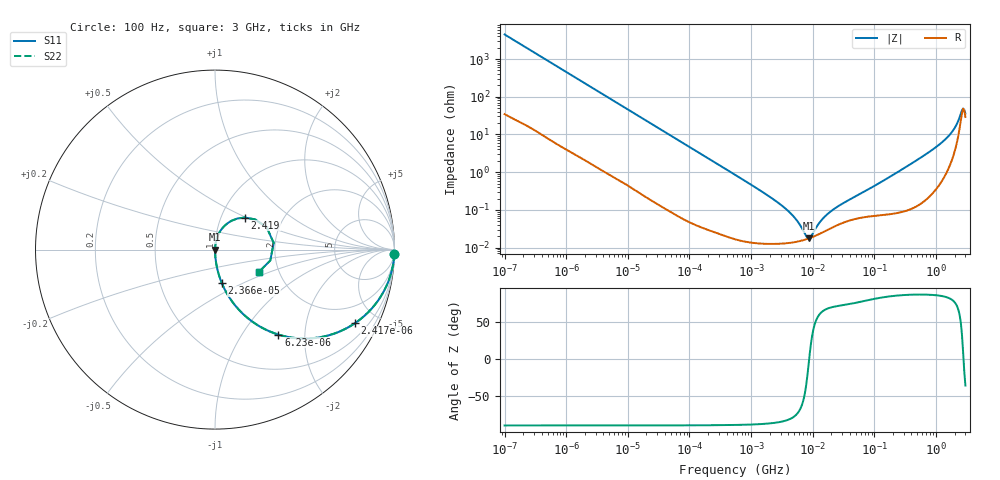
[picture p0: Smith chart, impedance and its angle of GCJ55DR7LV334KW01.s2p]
!Murata Part Number: GCJ55DR7LV334KW01
!These Parameters are Measured in Series Mode Connection
!Data Generated on Mar 13, 2026
!  o--ll--o
!Port1  Port2
!  o------o
!Operation Temp=25[degC], DC Bias Voltage=0[V]
!Freq. Start=100[Hz] Stop=3[GHz] 401[Steps]
# Hz S RI R 50
!Freq.(Hz) S11(Real) S11(Imag) S21(Real) S21(Imag) S12(Real) S12(Imag) S22(Real) S22(Imag)
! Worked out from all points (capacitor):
!   401 points, 100 Hz to 3 GHz, reference 50 ohm
!   read as one part in series: C = 354 nF near 109 Hz
!   lowest |Z| = 17.6 mohm at 8.608 MHz (marker M1)
!   series resonance near 8.758 MHz, so ESL is about 930 pH
!   S11 on the Smith chart (normalised r, x): 100 Hz: 2, -90; 2.417 kHz: 1.03, -3.78; 6.23 kHz: 1.01, -1.47; 23.66 kHz: 1.00, -0.39; 2.419 GHz: 1.29, +0.49; 3 GHz: 1.58, -0.42
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100  0.9993 -0.0223  0.000668 0.0223  0.000668 0.0223  0.9993 -0.0223
536  0.9852 -0.1164  0.0148 0.1164  0.0148 0.1164  0.9852 -0.1164
1788  0.8645 -0.3378  0.1355 0.3378  0.1355 0.3378  0.8645 -0.3378
2417  0.7792 -0.4102  0.2208 0.4102  0.2208 0.4102  0.7792 -0.4102
4051  0.5607 -0.4917  0.4393 0.4917  0.4393 0.4917  0.5607 -0.4917
6230  0.3535 -0.4733  0.6465 0.4733  0.6465 0.4733  0.3535 -0.4733
11382  0.1434 -0.3458  0.8566 0.3458  0.8566 0.3458  0.1434 -0.3458
23658  0.0385 -0.1879  0.9615 0.1879  0.9615 0.1879  0.0385 -0.1879
31977  0.0219 -0.1417  0.9781 0.1417  0.9781 0.1417  0.0219 -0.1417
547723  0.00024 -0.00856  0.9998 0.00856  0.9998 0.00856  0.00024 -0.00856
3486191  0.00013 -0.00113  0.9999 0.00113  0.9999 0.00113  0.00013 -0.00113
5135543  0.00014 -0.000595  0.9999 0.000595  0.9999 0.000595  0.00014 -0.000595
8607956  0.000175 -1.78e-05  0.9998 1.78e-05  0.9998 1.78e-05  0.000175 -1.78e-05
9794414  0.00019 0.000116  0.9998 -0.000116  0.9998 -0.000116  0.00019 0.000116
1.382041e7  0.000244 0.000472  0.9998 -0.000472  0.9998 -0.000472  0.000244 0.000472
2.035898e7  0.000336 0.000896  0.9997 -0.000896  0.9997 -0.000896  0.000336 0.000896
1.751444e8  0.00082 0.00736  0.9992 -0.00736  0.9992 -0.00736  0.00082 0.00736
1.163803e9  0.00796 0.0552  0.992 -0.0552  0.992 -0.0552  0.00796 0.0552
1.950712e9  0.0455 0.1245  0.9545 -0.1245  0.9545 -0.1245  0.0455 0.1245
2.419119e9  0.1666 0.1788  0.8334 -0.1788  0.8334 -0.1788  0.1666 0.1788
2.636591e9  0.2883 0.1237  0.7117 -0.1237  0.7117 -0.1237  0.2883 0.1237
3e9  0.2458 -0.1231  0.7542 0.1231  0.7542 0.1231  0.2458 -0.1231
